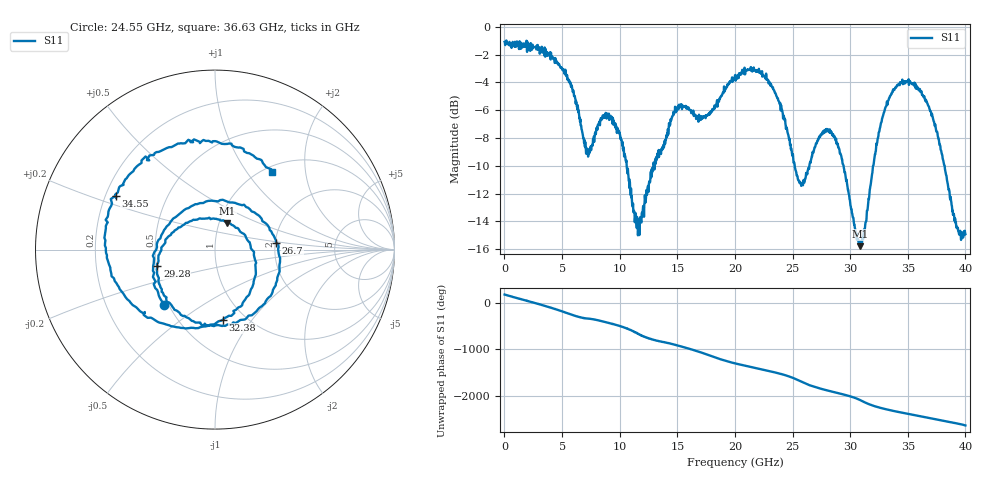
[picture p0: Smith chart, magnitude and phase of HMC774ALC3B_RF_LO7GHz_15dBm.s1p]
! Analog Devices, Inc.
! 1 Analog Way
! Wilmington, MA 01887
! http://www.analog.com
! Date:  2021-09-17 NN
! Board Name:  EV1HMC774ALC3B Revision A with HMC774ALC3B installed
! File Description:  S-Parameters for evaluation board without connectors or board loss de-embedded
! File Generation:  Calibrated Network Analyzer
! Chip Part Number:  HMC774ALC3B
! Chip Description:  MMIC, Double Balanced Mixer
! Chip Frequency:  7 to 34 GHz
! Chip Package:  LCC, 2.9 x 2.9 x 0.8 mm
! Chip State:
!  Temperature:  25C
!  LO Frequency:  7GHz
!  LO Power:  15dBm
! Note:
!  Analog Devices supplies this data as a sample of measured data at the evaluation board
!  ports for this product.  Your particular data for this product may vary.
!  Analog Devices reserves the right to change this data at anytime.
!  All lines below in this file are as is from the Network Analyzer.
!Keysight Technologies,N5245A,MY49151104,A.10.65.16
!Date: Thursday, August 05, 2021 14:43:28
!Correction: S11(Full 2 Port(1,2))
!S1P File: Measurement: S11:
# Hz S  dB  R 50
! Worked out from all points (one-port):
!   1601 points, 10 MHz to 40 GHz, reference 50 ohm
!   lowest |S11| = -15.8 dB at 30.88 GHz (marker M1), VSWR 1.39, Z = 54.7 + j16.6 ohm
!   |S11| at or under -10 dB: 10.6 GHz to 12.92 GHz (2.314 GHz wide, 19.7 % of centre); 29.43 GHz to 31.99 GHz (2.566 GHz wide, 8.36 % of centre); 38.2 GHz to end of sweep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
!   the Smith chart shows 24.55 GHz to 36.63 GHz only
!   S11 on the Smith chart (normalised r, x): 24.55 GHz: 0.47, -0.35; 26.7 GHz: 2.02, +0.18; 29.28 GHz: 0.51, -0.10; 32.38 GHz: 0.79, -0.73; 34.55 GHz: 0.24, +0.24; 36.63 GHz: 1.09, +1.33
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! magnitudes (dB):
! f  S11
! 10 MHz  -1.1
! 5.009 GHz  -3.0
! 5.934 GHz  -4.7
! 7.183 GHz  -9.0
! 8.708 GHz  -6.5
! 10.01 GHz  -7.8
! 11.68 GHz  -14.1
! 12.88 GHz  -10.1
! 15.01 GHz  -5.8
! 17.53 GHz  -6.4
! 20 GHz  -3.5
! 22.53 GHz  -3.6
! 24.55 GHz  -7.6
! 25 GHz  -9.3
! 25.8 GHz  -11.2
! 26.7 GHz  -9.3
! 28.05 GHz  -7.5
! 29.28 GHz  -9.5
! 30 GHz  -12.7
! 30.88 GHz  -15.8
! 32.38 GHz  -8.1
! 33.38 GHz  -5.1
! 34.55 GHz  -4.0
! 35 GHz  -3.9
! 36.63 GHz  -5.4
! 37.58 GHz  -7.7
! 39.25 GHz  -14.5
! 40 GHz  -14.9
